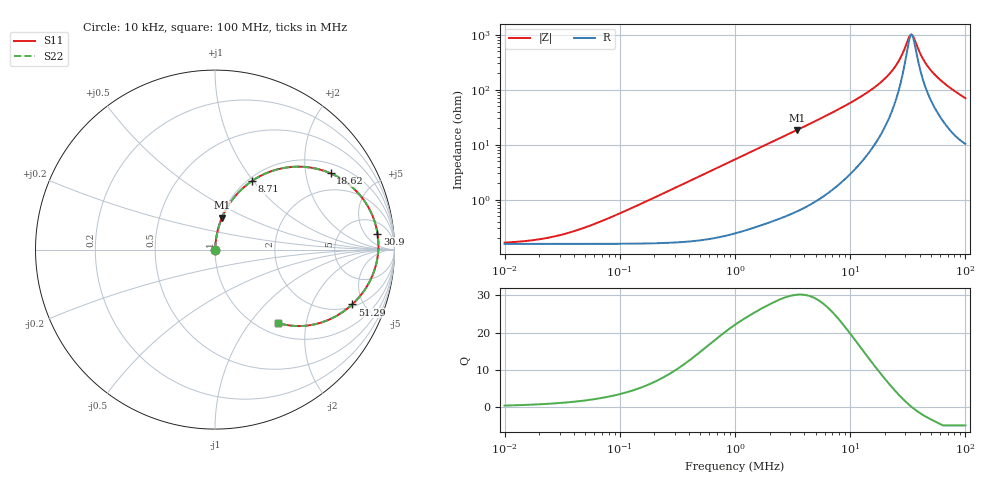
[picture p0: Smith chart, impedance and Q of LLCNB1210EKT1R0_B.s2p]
! LLCNB1210EKT1R0_B  S-PARAMETER MODEL  ( Standard Model )
! Model Generated by TAIYO YUDEN Corporation (http://www.ty-top.com)
! Version 1.0
! TAIYO YUDEN Control No. 191108
! Copyright(c) 2019 TAIYO YUDEN CO.,LTD. All Rights Reserved.
! Product Description (link to TY-COMPAS)
! https://ds.yuden.co.jp/TYCOMPAS/or/detail?pn=LLCNB1210EKT1R0MB&u=M
! Products Name : Inductors
! Characteristics :
!  Inductance : 1.0 [uH] , SRF(min) : - [Hz] , DC Resistance(max) : 179 [mOhm]
!  Rated Current : Saturation  1.5 [A] (dL = 30 [%]), Temp Rise  1.1 [A] (dT = 40 [degC])
!  Case Size : 1.25 x 1.05 / 0.049 x 0.041 [mm/inch] , Thickness : 0.5 / 0.02 [mm/inch]
!  (Conditions: Temperature = 25 [degC] , DC Bias Current = 0 [A])
! External Node Assignments :
!  1  o---GGG---o  2
! GND o---------o GND
! Frequency Range : 10kHz  -  100MHz  [ 402 STEP ]
# MHz S RI R 50
! Freq[MHz].  S11 Real  S11 Imag  S21 Real  S21 Imag  S12 Real  S12 Imag  S22 Real  S22 Imag
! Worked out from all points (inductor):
!   401 points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, 10 kHz to 100 MHz, reference 50 ohm
!   read as one part in series: L = 862 nH near 89.12 kHz
!   highest Q = 30.2 at 3.467 MHz (marker M1), where L = 852 nH
!   self-resonance near 34.1 MHz
!   S11 on the Smith chart (normalised r, x): 10 kHz: 1.00, +0.00; 8.71 MHz: 1.04, +0.98; 18.62 MHz: 1.32, +2.76; 30.9 MHz: 10, +11; 51.29 MHz: 2.17, -4.10; 100 MHz: 1.21, -1.39
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0.01  0.00157 0.00054  0.9984 -0.00054  0.9984 -0.00054  0.00157 0.00054
0.022387  0.00157 0.00121  0.9984 -0.00121  0.9984 -0.00121  0.00157 0.00121
0.046774  0.00158 0.00253  0.9984 -0.00253  0.9984 -0.00253  0.00158 0.00253
0.087096  0.0016 0.0047  0.9984 -0.0047  0.9984 -0.0047  0.0016 0.0047
0.218776  0.00176 0.0118  0.9982 -0.0118  0.9982 -0.0118  0.00176 0.0118
1  0.0053 0.0534  0.9947 -0.0534  0.9947 -0.0534  0.0053 0.0534
3.467369  0.0388 0.1773  0.9612 -0.1773  0.9612 -0.1773  0.0388 0.1773
4.677351  0.0667 0.2331  0.9333 -0.2331  0.9333 -0.2331  0.0667 0.2331
6.606934  0.1251 0.3124  0.8749 -0.3124  0.8749 -0.3124  0.1251 0.3124
8.709636  0.2049 0.3816  0.7951 -0.3816  0.7951 -0.3816  0.2049 0.3816
13.48963  0.4199 0.4599  0.5801 -0.4599  0.5801 -0.4599  0.4199 0.4599
18.62087  0.6437 0.425  0.3563 -0.425  0.3563 -0.425  0.6437 0.425
21.87762  0.756 0.3552  0.244 -0.3552  0.244 -0.3552  0.756 0.3552
26.30268  0.8582 0.2293  0.1418 -0.2293  0.1418 -0.2293  0.8582 0.2293
28.18383  0.8841 0.1717  0.1159 -0.1717  0.1159 -0.1717  0.8841 0.1717
30.90295  0.9053 0.0897  0.0947 -0.0897  0.0947 -0.0897  0.9053 0.0897
33.11311  0.9105 0.0264  0.0895 -0.0264  0.0895 -0.0264  0.9105 0.0264
34.67368  0.9088 -0.0155  0.0912 0.0155  0.0912 0.0155  0.9088 -0.0155
42.65795  0.8558 -0.1887  0.1442 0.1887  0.1442 0.1887  0.8558 -0.1887
51.28614  0.764 -0.3056  0.236 0.3056  0.236 0.3056  0.764 -0.3056
70.79458  0.5603 -0.4153  0.4397 0.4153  0.4397 0.4153  0.5603 -0.4153
100  0.3512 -0.4086  0.6488 0.4086  0.6488 0.4086  0.3512 -0.4086
